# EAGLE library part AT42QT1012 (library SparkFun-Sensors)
One channel capacitive touch sense
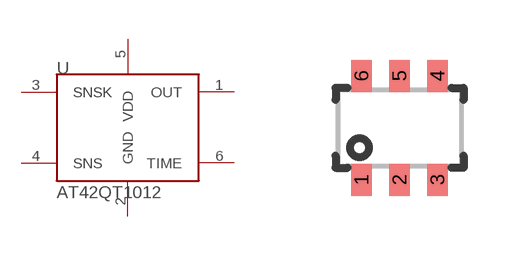
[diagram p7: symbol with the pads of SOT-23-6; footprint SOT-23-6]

Designator prefix U

## AT42QT1012  [SOT-23-6]
1  OUT
2  GND
3  SNSK
4  SNS
5  VDD
6  TIME

## Footprint SOT-23-6 (pad centres in mm)
smd 0.51 x 0.8: 1 -0.95,-1.3; 2 0,-1.3; 3 0.95,-1.3; 4 0.95,1.3; 5 0,1.3; 6 -0.95,1.3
